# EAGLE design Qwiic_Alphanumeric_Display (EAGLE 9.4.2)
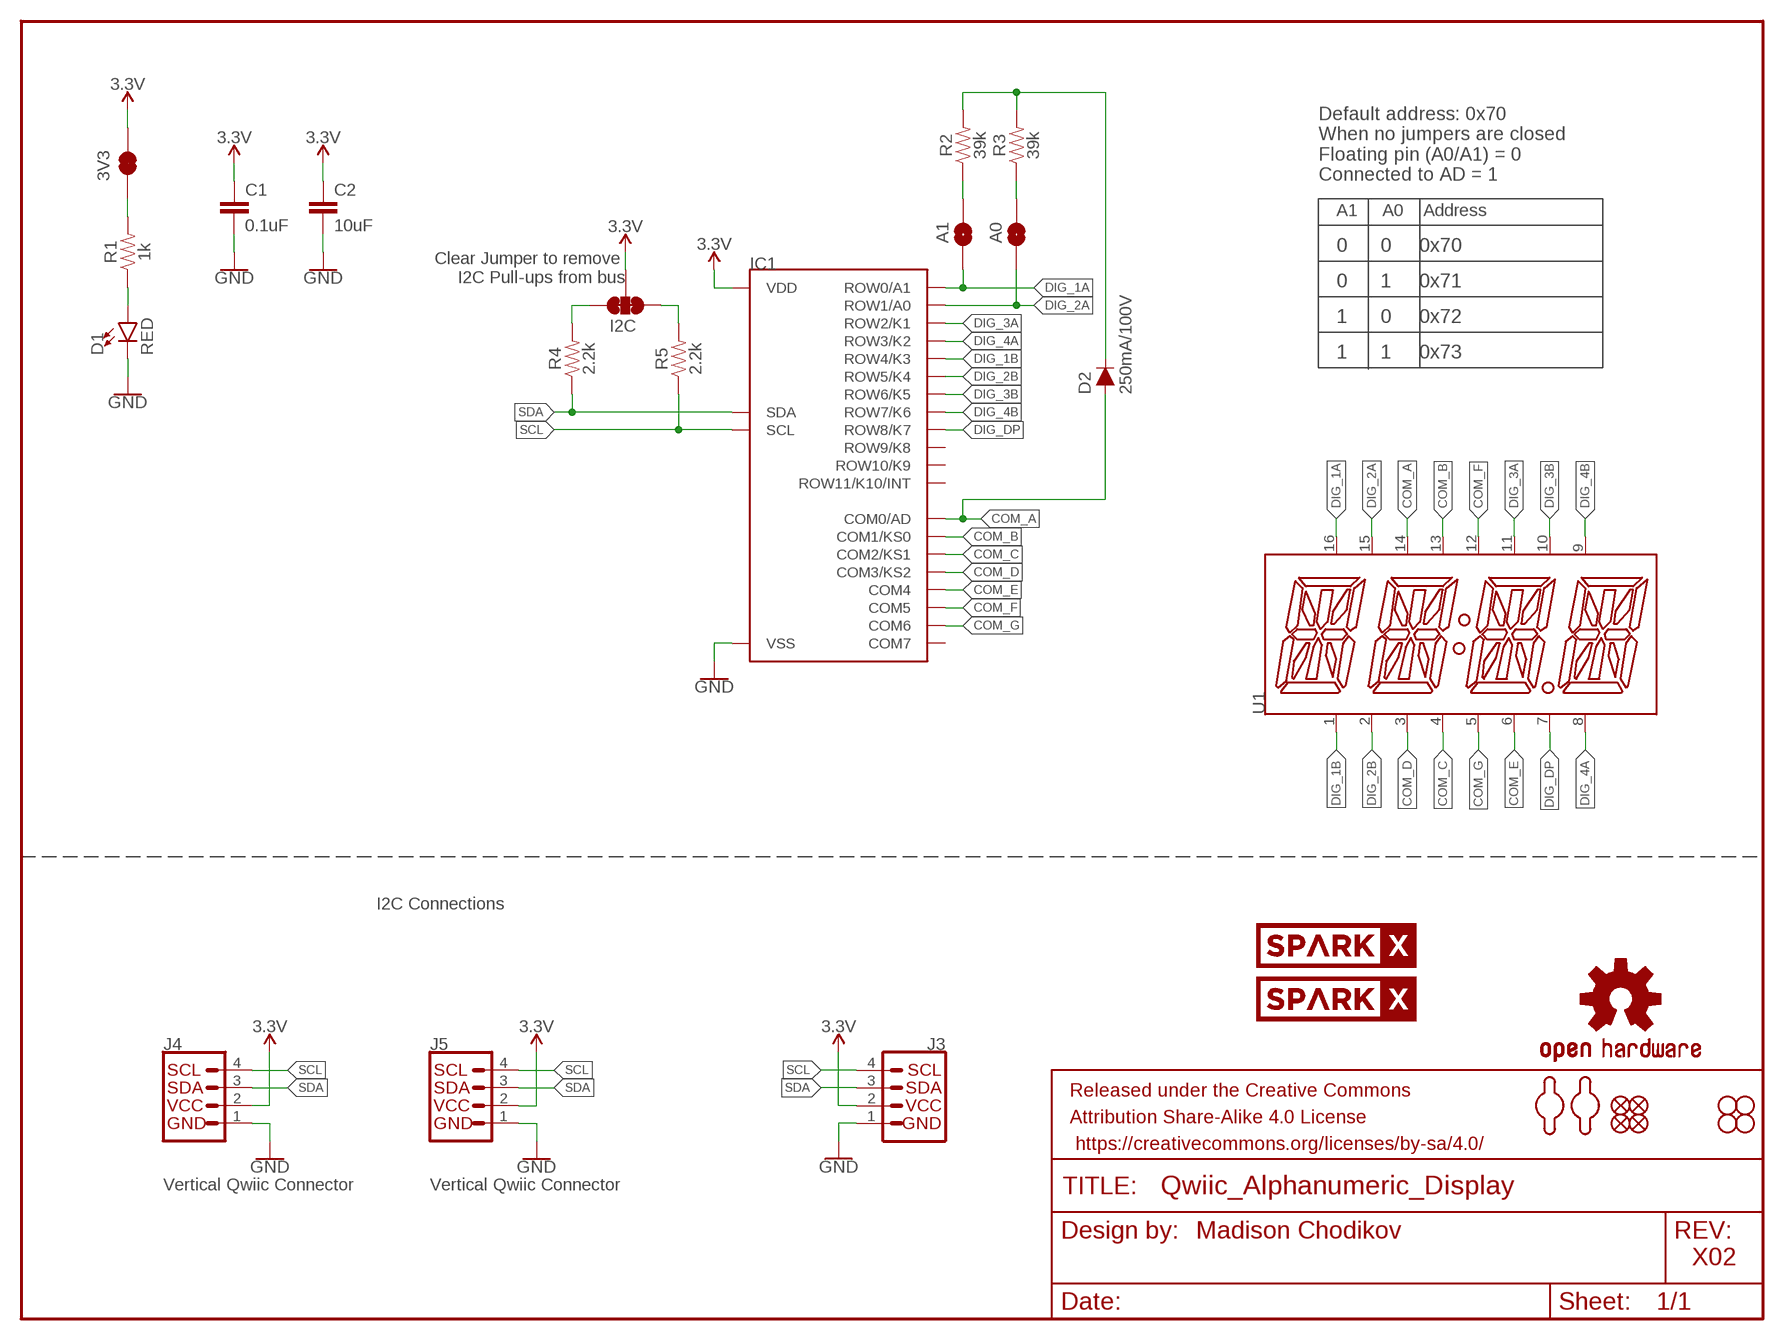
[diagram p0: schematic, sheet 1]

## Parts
3V3  JUMPER-SMT_2_NC_TRACE_SILK  [SMT-JUMPER_2_NC_TRACE_SILK]
A0  JUMPER-SMT_2_NO_SILK  [SMT-JUMPER_2_NO_SILK]
A1  JUMPER-SMT_2_NO_SILK  [SMT-JUMPER_2_NO_SILK]
C1  0.1uF  0.1UF-0603-25V-5%  [0603]
C2  10uF  10UF-0603-6.3V-20%  [0603]
D1  RED  LED-RED0603  [LED-0603]
D2  250mA/100V  DIODE-BAS16J  [SOD-323]
FD1  FIDUCIAL1X2  [FIDUCIAL-1X2]
FD2  FIDUCIAL1X2  [FIDUCIAL-1X2]
FD3  FIDUCIAL1X2  [FIDUCIAL-1X2]
FD4  FIDUCIAL1X2  [FIDUCIAL-1X2]
FRAME1  FRAME-LETTER  [CREATIVE_COMMONS]
H1  STAND-OFF  [STAND-OFF]
H2  STAND-OFF  [STAND-OFF]
H3  STAND-OFF  [STAND-OFF]
H4  STAND-OFF  [STAND-OFF]
I2C  JUMPER-SMT_3_2-NC_TRACE_SILK  [SMT-JUMPER_3_2-NC_TRACE_SILK]
IC1  HT16K33  [HT16K33]
J3  I2C_STANDARD_NO_SILK  [1X04_NO_SILK]
J4  Vertical Qwiic Connector  QWIIC_CONNECTOR  [JST04_1MM_VERT]
J5  Vertical Qwiic Connector  QWIIC_CONNECTOR  [JST04_1MM_VERT]
LOGO1  OSHW-LOGOMINI  [OSHW-LOGO-MINI]
R1  1k  1KOHM-0603-1/10W-1%  [0603]
R2  39k  39KOHM-0603-1/10W-1%  [0603]
R3  39k  39KOHM-0603-1/10W-1%  [0603]
R4  2.2k  2.2KOHM-0603-1/10W-1%  [0603]
R5  2.2k  2.2KOHM-0603-1/10W-1%  [0603]
U1  SILSMART_DISPLAY  [SILSMART_DISPLAY]
U$7  SPARKX-LOGO4  [SPARKX-MEDIUM]
U$8  SPARKX-LOGO4  [SPARKX-MEDIUM]
U$18  MOUNTING_HOLE_M2-0.4X6  [MOUNTING_HOLE_M2-0.4X6]
U$19  MOUNTING_HOLE_M2-0.4X6  [MOUNTING_HOLE_M2-0.4X6]

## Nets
3.3V: 3V3.2 C1.1 C2.1 I2C.2 IC1.24(VDD) J3.2 J4.2 J5.2
COM_A: D2.A IC1.2(COM0/AD) U1.14(COM_A)
COM_B: IC1.3(COM1/KS0) U1.13(COM_B)
COM_C: IC1.4(COM2/KS1) U1.4(COM_C)
COM_D: IC1.5(COM3/KS2) U1.3(COM_D)
COM_E: IC1.6(COM4) U1.6(COM_E)
COM_F: IC1.7(COM5) U1.12(COM_F)
COM_G: IC1.8(COM6) U1.5(COM_G1)
DIG_1A: A1.1 IC1.21(ROW0/A1) U1.16(DIG_1A)
DIG_1B: IC1.17(ROW4/K3) U1.1(DIG_1B)
DIG_2A: A0.1 IC1.20(ROW1/A0) U1.15(DIG_2A)
DIG_2B: IC1.16(ROW5/K4) U1.2(DIG_2B)
DIG_3A: IC1.19(ROW2/K1) U1.11(DIG_3A)
DIG_3B: IC1.15(ROW6/K5) U1.10(DIG_3B)
DIG_4A: IC1.18(ROW3/K2) U1.8(DIG_4A)
DIG_4B: IC1.14(ROW7/K6) U1.9(DIG_4B)
DIG_DP: IC1.13(ROW8/K7) U1.7(DIG_DP)
GND: C1.2 C2.2 D1.C IC1.1(VSS) J3.1 J4.1 J5.1
N$1: D1.A R1.1
N$2: A1.2 R2.1
N$3: A0.2 R3.1
N$4: I2C.1 R5.2
N$5: I2C.3 R4.2
N$6: D2.C R2.2 R3.2
N$7: 3V3.1 R1.2
SCL: IC1.22(SCL) J3.4 J4.4 J5.4 R5.1
SDA: IC1.23(SDA) J3.3 J4.3 J5.3 R4.1
Unconnected: IC1.9(COM7) IC1.10(ROW11/K10/INT) IC1.11(ROW10/K9) IC1.12(ROW9/K8)

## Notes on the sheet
- Default address: 0x70
  When no jumpers are closed
  Floating pin (A0/A1) = 0
  Connected to AD = 1
- A1     A0    Address
- Clear Jumper to remove 
  I2C Pull-ups from bus
- 0      0     0x70
- 0      1     0x71
- 1      0     0x72
- 1      1     0x73
- I2C Connections
- Madison Chodikov
- X02

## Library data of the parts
3V3 = SparkFun-Jumpers:JUMPER-SMT_2_NC_TRACE: Normally closed trace jumper
A0 A1 = SparkFun-Jumpers:JUMPER-SMT_2_NO: Normally open jumper
C1 = SparkFun-Capacitors:0.1UF: 0.1µF ceramic capacitors; PROD_ID: CAP-08604
C2 = SparkFun-Capacitors:10UF: 10.0µF ceramic capacitors; PROD_ID: CAP-11015
D1 = SparkFun-LED:LED-RED: Red SMD LED; PROD_ID: DIO-00819
D2 = SparkFun-DiscreteSemi:DIODE: Diode; PROD_ID: DIO-09646
FD1-FD4 = SparkFun-Aesthetics:FIDUCIAL: Fiducial Alignment Points
FRAME1 = SparkFun-Aesthetics:FRAME-LETTER: Schematic Frame - Letter
H1-H4 = SparkFun-Hardware:STAND-OFF: Stand Off
I2C = SparkFun-Jumpers:JUMPER-SMT_3_2-NC_TRACE: Normally closed trace jumper (2 of 2 connections) This jumper has a trace between all three pads so they are normally closed (NC). Use a razor knife to open the connection(s). For best results follow the IPC guidelines for cutting traces: Cutout at least 0.063 mm (0.005 in). Remove all loose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
IC1 = Alphanumeric_Display_Library:HT16K33: HT16K33 24 SOP-A : RAM Mapping 16x8 LED Controller Driver with Keyscan; PROD_ID: IC-14891
J3 = SparkFun-Connectors:I2C_STANDARD: SparkFun I2C Standard Pinout Header SparkFun has standardized on a pinout for all I2C based sensor breakouts. This pinout allows I2C boards to be plugged directly into the headers on Arduino Uno compatible boards, and to be daisy chained easily. Example SparkFun Products: SparkFun Atmospheric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
J4 J5 = SparkFun-Connectors:QWIIC_CONNECTOR: SparkFun I2C Standard Qwiic Connector An SMD 1mm pitch JST connector makes it easy and quick (get it? Qwiic?) to connect I2C devices to each other. The Qwiic system enables fast and solderless connection between popular platforms and various sensors and actuators. We carry 200mm, 100mm, 50mm, and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; PROD_ID: CONN-14483
LOGO1 = SparkFun-Aesthetics:OSHW-LOGO: Open-Source Hardware (OSHW) Logo
R1 = SparkFun-Resistors:1KOHM: 1kΩ resistor; PROD_ID: RES-07856
R2 R3 = SparkFun-Resistors:39KOHM: 39kΩ resistor; PROD_ID: RES-12377
R4 R5 = SparkFun-Resistors:2.2KOHM: 2.2kΩ resistor; PROD_ID: RES-08272
U1 = Alphanumeric_Display_Library:SILSMART_DISPLAY: 14-Segment Alphanumeric LED Display from Silsmart Optoelectronics; PROD_ID: COMP-14892
U$7 U$8 = SparkX:SPARKX-LOGO
U$18 U$19 = Alphanumeric_Display_Library:MOUNTING_HOLE_M2-0.4X6

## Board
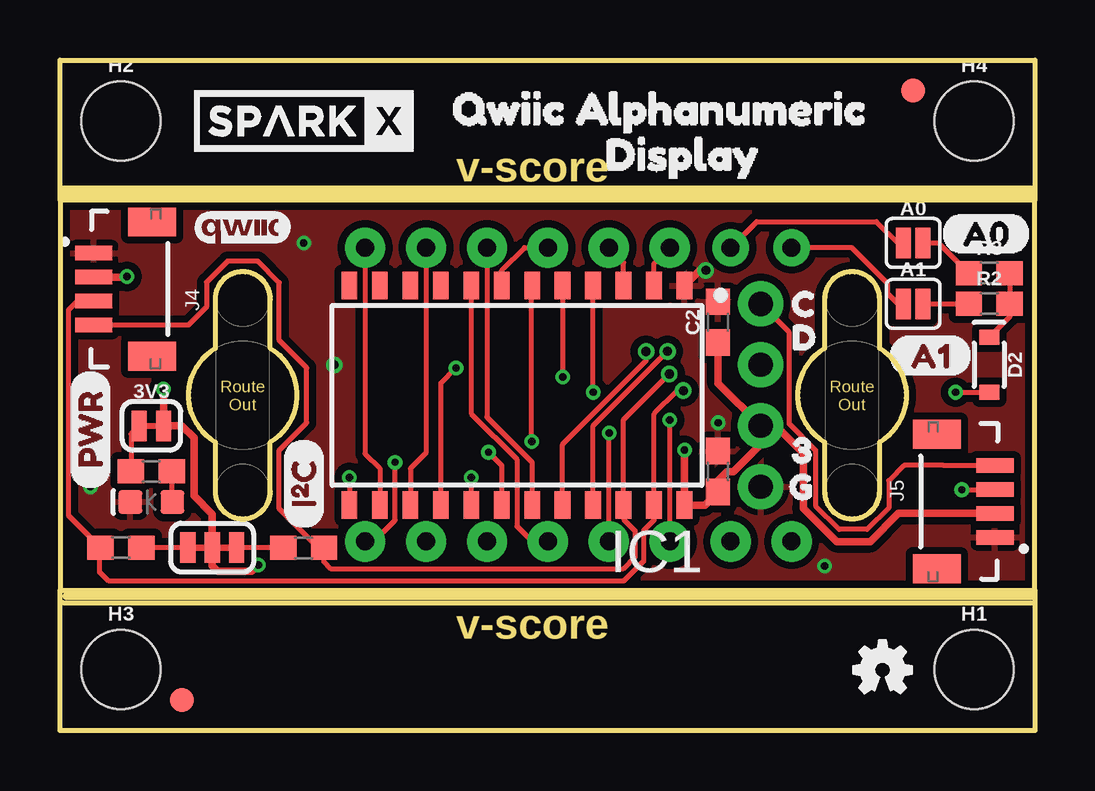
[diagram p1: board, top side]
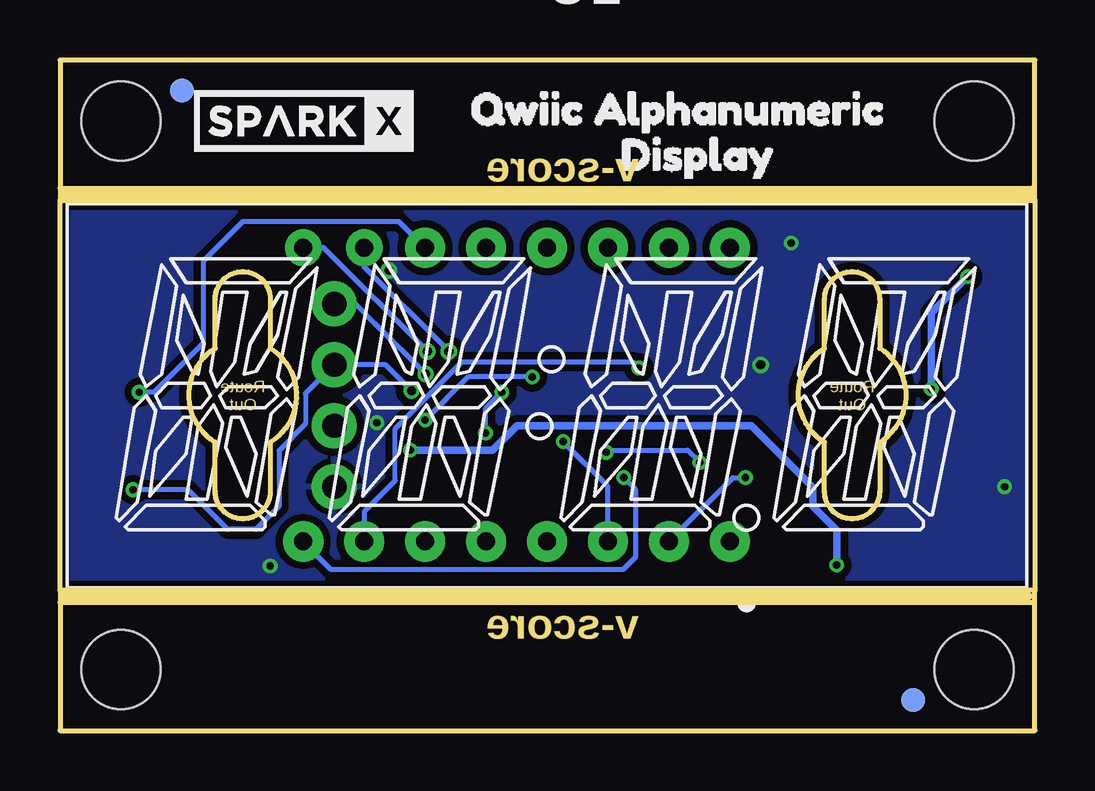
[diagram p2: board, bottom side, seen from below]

Size 40.64 x 27.94 mm. Coordinates in mm from the lower left corner, seen from the top.
Outline: 0,5.84 40.64,5.84
Outline: 40.64,5.84 40.64,22.1
Outline: 40.64,22.1 0,22.1
Outline: 0,22.1 0,5.84
Outline: 0,22.1 0,27.94 40.64,27.94 40.64,22.1
Outline: 40.64,5.84 40.64,0 0,0 0,5.84
Outline: 40.64,22.61 0.13,22.61
Outline: 0.13,5.33 40.64,5.33
Copper layers (1*16): Top 0.035mm / dielectric 1.5mm / Bottom 0.035mm
Design rules "SparkFun-2-layer-PCBWay-LIMIT": minimum track width 6mil, minimum drill 0.3mm, track to track 6mil, track to pad 6mil, pad to pad 6mil, via to via 6mil, smd to smd 6mil, copper to edge 6mil, drill to drill 6mil, minimum pad ring 6mil, minimum via ring 6mil, stop-mask expansion 4mil, vias tented up to drill 25mil, thermal gap 10mil
Milling: 2 lines

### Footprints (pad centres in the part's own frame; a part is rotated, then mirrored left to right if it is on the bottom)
SMT-JUMPER_2_NC_TRACE_SILK = smd 0.635 x 1.27: 1 -0.508,0; 2 0.508,0
SMT-JUMPER_2_NO_SILK = smd 0.635 x 1.27: 1 -0.406,0; 2 0.406,0
0603 = smd 1.1 x 1: 1 -0.85,0; 2 0.85,0
LED-0603 = smd 1 x 1: A -0.877,0; C 0.877,0
SOD-323 = smd 0.63 x 0.83: A 1.15,0; C -1.15,0
FIDUCIAL-1X2 = smd 1 x 1: 1 0,0
STAND-OFF = hole 3.302: 0,0
SMT-JUMPER_3_2-NC_TRACE_SILK = smd 0.635 x 1.27: 1 -1.016,0; 2 0,0; 3 1.016,0
HT16K33 = smd 0.66 x 1.143: 1 -6.985,-4.572; 2 -5.715,-4.572; 3 -4.445,-4.572; 4 -3.175,-4.572; 5 -1.905,-4.572; 6 -0.635,-4.572; 7 0.635,-4.572; 8 1.905,-4.572; 9 3.175,-4.572; 10 4.445,-4.572; 11 5.715,-4.572; 12 6.985,-4.572; 13 6.985,4.572; 14 5.715,4.572; 15 4.445,4.572; 16 3.175,4.572; 17 1.905,4.572; 18 0.635,4.572; 19 -0.635,4.572; 20 -1.905,4.572; 21 -3.175,4.572; 22 -4.445,4.572; 23 -5.715,4.572; 24 -6.985,4.572
1X04_NO_SILK = drill 1.016 pad 1.88: 1 0,0; 2 2.54,0; 3 5.08,0; 4 7.62,0
JST04_1MM_VERT = smd 0.6 x 1.55: 1 -1.478,0.775; 2 -0.478,0.775; 3 0.522,0.775; 4 1.522,0.775 | smd 1.2 x 2: NC1 -2.778,3.2; NC2 2.822,3.2
SILSMART_DISPLAY = drill 0.75 pad 1.676: 1 -10.178,-6.092; 2 -7.638,-6.092; 3 -5.098,-6.092; 4 -2.558,-6.092; 5 -0.018,-6.092; 6 2.522,-6.092; 7 5.062,-6.092; 8 7.602,-6.092; 9 7.602,6.148; 10 5.062,6.148; 11 2.522,6.148; 12 -0.018,6.148; 13 -2.558,6.148; 14 -5.098,6.148 | drill 0.75 pad 1.524: 15 -7.638,6.148; 16 -10.178,6.148

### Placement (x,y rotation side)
3V3  3.81,12.7 0 top
A0  35.56,20.32 0 top
A1  35.56,17.78 0 top
C1  27.43,10.79 90 top
C2  27.43,17.02 90 top
D1  3.81,9.53 180 top
D2  38.73,15.24 270 top
FD1  5.08,1.27 0 top
FD2  5.08,1.27 0 bottom
FD3  35.56,26.67 0 top
FD4  35.56,26.67 0 bottom
FRAME1  not placed on the board
H1  38.1,2.54 0 top
H2  2.54,25.4 0 top
H3  2.54,2.54 0 top
H4  38.1,25.4 0 top
I2C  6.35,7.62 180 top
IC1  19.05,13.97 180 top
J3  29.21,10.16 90 top
J4  0.64,18.41 270 top
J5  39.75,9.53 90 top
LOGO1  34.29,2.54 0 top
R1  3.81,10.79 180 top
R2  38.73,17.78 0 top
R3  38.73,19.05 0 top
R4  2.54,7.62 0 top
R5  10.16,7.62 180 top
U1  20.32,13.97 0 bottom
U$1  [32]  29.59,11.68 0 top
U$2  [C0]  29.59,17.78 0 top
U$3  [PWR5]  1.27,10.03 90 top
U$4  [D1]  29.59,16.38 0 top
U$5  [G3]  29.46,10.16 0 top
U$6  [QWIIC_4MM]  7.62,20.96 0 top
U$7  10.16,25.4 0 top
U$8  30.48,25.4 0 bottom
U$10  [I_SUPER2_C-()-04]  10.16,8.38 90 top
U$13  [QWIIC_ALPHANUMERIC0]  24.64,25.91 0 bottom
U$15  [QWIIC_ALPHANUMERIC0]  15.24,25.91 0 top
U$16  [DISPLAY1]  21.59,24 0 top
U$17  [DISPLAY1]  18.41,24 0 bottom
U$18  33.02,13.97 0 top
U$19  7.62,13.97 0 top
U$20  [A00]  36.7,20.7 0 top
U$21  [A11]  34.54,15.62 0 top

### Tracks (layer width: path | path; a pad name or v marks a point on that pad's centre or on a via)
3.3V  (via drill 0.3)
  Top 0.203: 2.76,18.89 v2.79,18.92
  Top 0.305: J3.2 29.84,12.7 30.99,11.56 30.99,9.27 32.38,7.87 33.78,7.87 34.95,9.05 J5.2 | v26.04,11.68 IC1.24 26.89,9.4 C1.1 27.43,10.41 27.81,10.79 28.08,10.79 29.21,11.92 J3.2 | J4.2 2.76,18.89 | v4.32,14.22 3V3.2 5.08,12.7 5.59,12.19 5.59,9.78 6.35,9.02 I2C.2 6.35,6.86 6.58,6.63 8,6.63 v8.27,6.9 | J3.2 27.43,14.48 C2.1
  Bottom 0.305: v26.04,11.68 22.61,11.68 21.59,12.7 11.81,12.7 9.25,10.14 9.25,9.34 8.27,8.35 v8.27,6.9 | v2.79,18.92 4.32,17.4 v4.32,14.22
COM_A  (via drill 0.3)
  Top 0.203: v37.34,14.1 D2.A | IC1.2 24.77,19.46 U1.14
  Bottom 0.203: U1.14 26.51,21.21 33.02,21.21 34.67,19.56 34.67,16.13 36.7,14.1 v37.34,14.1
COM_B
  Top 0.203: IC1.3 23.5,19.5 U1.13
COM_C  (via drill 0.3)
  Top 0.203: v22.23,14.1 IC1.4 | U1.4 22.88,12.38 v22.9,12.4
  Bottom 0.203: v22.9,12.4 22.9,13.42 v22.23,14.1
COM_D  (via drill 0.3)
  Top 0.203: IC1.5 v20.95,14.73 | U1.3 v25.42,12.94
  Bottom 0.203: v20.95,14.73 23.62,14.73 v25.42,12.94
COM_E  (via drill 0.3)
  Top 0.203: v19.66,12.04 19.66,18.52 IC1.6
  Bottom 0.203: U1.6 17.8,10.18 v19.66,12.04
COM_F
  Top 0.203: IC1.7 18.41,19.18 19.36,20.12 U1.12
COM_G
  Top 0.203: IC1.8 17.14,13.21 19.05,11.3 19.05,8.51 19.68,7.88 U1.5
DIG_1A  (via drill 0.38)
  Top 0.203: A1.1 34.92,17.78 34.51,18.2 34.51,18.62 33.01,20.12 U1.16 | IC1.21 22.23,12.7 v25.32,15.8
  Bottom 0.203: v25.32,15.8 29.64,20.12 U1.16
DIG_1B  (via drill 0.3)
  Top 0.203: v17.14,10.54 IC1.17
  Bottom 0.203: U1.1 29.35,6.73 17.14,6.73 16.64,7.24 16.64,10.03 v17.14,10.54
DIG_2A  (via drill 0.38)
  Top 0.203: U1.15 29.05,21.21 34.04,21.21 34.92,20.32 A0.1 | IC1.20 20.95,11.94 24.43,15.41 v24.43,15.79
  Bottom 0.203: v24.43,15.79 27.96,19.32 U1.15
DIG_2B  (via drill 0.3)
  Top 0.203: IC1.16 15.88,14.48 v16.51,15.11
  Bottom 0.203: v16.51,15.11 16.76,15.37 23.88,15.37 26.67,12.57 26.67,10.41 27.94,9.14 27.94,7.9 U1.2
DIG_3A
  Top 0.203: U1.11 17.8,13.06 19.68,11.18 IC1.19
DIG_3B
  Top 0.203: U1.10 15.26,11.58 14.61,10.92 IC1.15
DIG_4A  (via drill 0.3)
  Top 0.203: U1.8 13.09,7.88 13.97,8.76 v13.97,11.18 | v17.87,11.6 18.41,11.05 IC1.18
  Bottom 0.203: v13.97,11.18 14.48,11.68 17.78,11.68 v17.87,11.6
DIG_4B
  Top 0.203: U1.9 12.72,11.54 13.34,10.92 IC1.14
DIG_DP  (via drill 0.3)
  Top 0.203: v12.06,10.54 IC1.13
  Bottom 0.203: U1.7 12.6,10.54 v12.06,10.54
GND  (via drill 0.3, 0.38)
  Top 0.305: IC1.1 26.67,19.18 v26.92,19.18
  other vias: 10.16,20.32 27.43,12.83 1.27,10.16 31.88,6.86 11.43,15.24
  pour Top (isolate 0.305): 0,5.84 0,22.1 40.64,22.1 40.64,5.84
  pour Bottom (isolate 0.305): 0,22.1 40.64,22.1 40.64,5.84 0,5.84
N$1
  Top 0.203: D1.A 4.69,10.77 R1.1
N$2
  Top 0.203: A1.2 R2.1
N$3
  Top 0.203: A0.2 36.62,20.32 R3.1
N$4
  Top 0.203: R5.2 I2C.1
N$5
  Top 0.203: I2C.3 R4.2
N$6
  Top 0.203: R3.2 R2.2 39.59,17.24 D2.C
N$7
  Top 0.203: 3V3.1 2.96,12.36 R1.2
SCL  (via drill 0.38)
  Top 0.203: J3.4 30.4,16.59 30.4,12.78 31.5,11.68 31.5,9.36 32.47,8.38 33.66,8.38 34.54,9.27 34.54,10.41 35.18,11.05 36.83,11.05 J5.4 | v25.4,14.86 23.5,12.95 IC1.22 23.5,8.81 23.97,8.33 23.97,7.24 23.46,6.73 11.3,6.73 11.01,7.02 R5.1 10.76,7.62 9.14,9.23 9.14,11.68 10.29,12.83 10.29,15.11 9.14,16.26 9.14,18.67 8.26,19.56 6.99,19.56 6.11,18.69 6.11,17.65 5.35,16.89 J4.4
  Bottom 0.203: v25.4,14.86 27.5,16.95 28.32,17.78 J3.4
SDA  (via drill 0.3, 0.38)
  Top 0.203: J5.3 38.96,10.03 v37.59,10.03 | J4.3 0.72,17.89 0.36,17.53 0.36,8.95 R4.1 1.65,7.58 1.65,6.6 2.03,6.22 23.5,6.22 24.33,7.05 24.33,8.33 24.77,8.77 IC1.23 24.77,13.2 25.73,14.16 v25.98,14.16
  Bottom 0.203: v37.59,10.03 35.31,10.03 33.66,8.38 32.47,8.38 31.51,9.34 31.51,11.67 30.4,12.78 30.4,14.05 J3.3 27.06,15.24 v25.98,14.16

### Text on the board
Dimension: v-score | v-score
tDocu: Madison Chodikov
_tNames: I2C
_bNames: U1

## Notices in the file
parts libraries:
SparkFun-Aesthetics: Licensing: Creative Commons ShareAlike 4.0 International - https://creativecommons.org/licenses/by-sa/4.0
SparkFun-Aesthetics: Released under the Creative Commons Attribution Share-Alike 4.0 License
SparkFun-Aesthetics: https://creativecommons.org/licenses/by-sa/4.0
